FUNCTION "CICLO FORMAZIONE PACCHI" : VOID
TITLE =CICLO AUTOMATICO FORMAZIONE PACCHI
VERSION : 0.1

BEGIN
NETWORK
TITLE =START CICLO
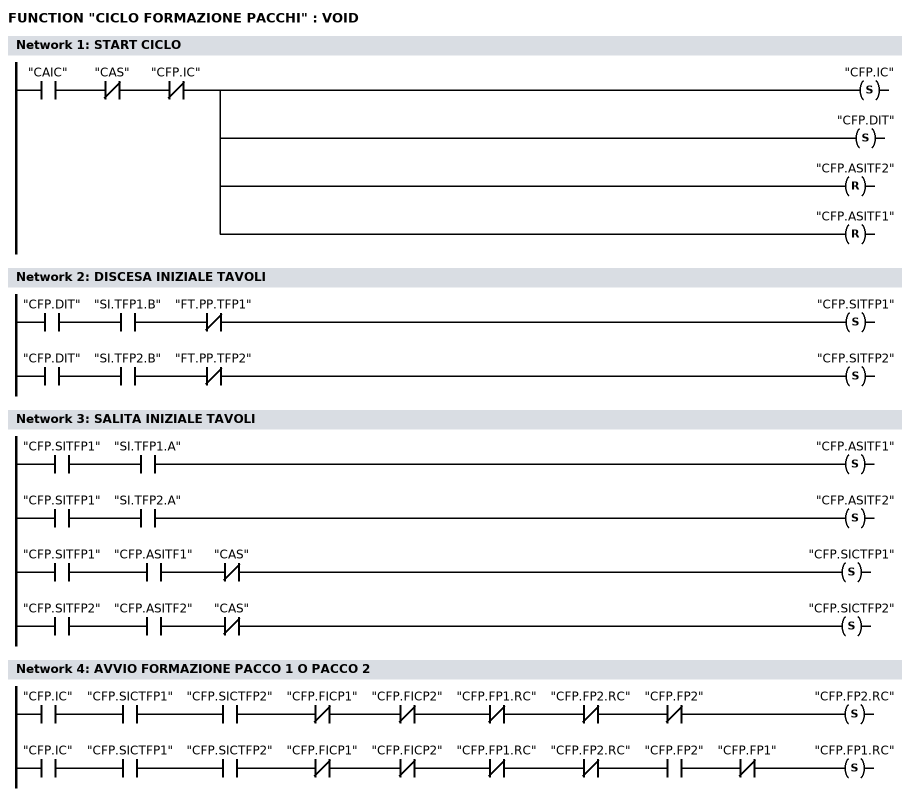
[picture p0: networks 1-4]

      U     "CAIC";
      UN    "CAS";
      UN    "CFP.IC";
      S     "CFP.IC";
      S     "CFP.DIT";
      R     "CFP.ASITF2";
      R     "CFP.ASITF1";
NETWORK
TITLE =DISCESA INIZIALE TAVOLI

      U     "CFP.DIT";
      U     "SI.TFP1.B";
      UN    "FT.PP.TFP1";
      S     "CFP.SITFP1";
//-----------------------------
      U     "CFP.DIT";
      U     "SI.TFP2.B";
      UN    "FT.PP.TFP2";
      S     "CFP.SITFP2";

NETWORK
TITLE =SALITA INIZIALE TAVOLI

      U     "CFP.SITFP1";
      U     "SI.TFP1.A";
      S     "CFP.ASITF1";
//---------------------------
      U     "CFP.SITFP1";
      U     "SI.TFP2.A";
      S     "CFP.ASITF2";
//====================================
      U     "CFP.SITFP1";
      U     "CFP.ASITF1";
      UN    "CAS";
      S     "CFP.SICTFP1";
//====================================
      U     "CFP.SITFP2";
      U     "CFP.ASITF2";
      UN    "CAS";
      S     "CFP.SICTFP2";

NETWORK
TITLE =AVVIO FORMAZIONE PACCO 1 O PACCO 2

      U     "CFP.IC";
      U     "CFP.SICTFP1";
      U     "CFP.SICTFP2";
      UN    "CFP.FICP1";
      UN    "CFP.FICP2";
      UN    "CFP.FP1.RC";
      UN    "CFP.FP2.RC";
      UN    "CFP.FP2";
      S     "CFP.FP2.RC";
//-----------------------
      U     "CFP.IC";
      U     "CFP.SICTFP1";
      U     "CFP.SICTFP2";
      UN    "CFP.FICP1";
      UN    "CFP.FICP2";
      UN    "CFP.FP1.RC";
      UN    "CFP.FP2.RC";
      U     "CFP.FP2";
      UN    "CFP.FP1";
      S     "CFP.FP1.RC";

NETWORK
TITLE =FORMAZIONE PACCO 2

//____________________________________
//      Inizio ciclo
//____________________________________
      U     "CFP.FP2.RC";
      UN    "CFP.FP2";
      S     "CFP.FP2";
      S     "CFP.FICP2";
      R     "CNP.FP2";
      R     "CFP.FP2.RC";
//____________________________________
//      Inibizione discesa tavolo
//____________________________________
      U     "CFP.FP2";
      U     "CFP.FICP2";
      U     "SI.PCA";
      S     "CFP.IDTF2";
      S     "CFP.CAP2";
//____________________________________
//      Discesa tavolo
//____________________________________
      U     "CFP.FP2";
      U     "CFP.FICP2";
      U     "FT.CLP.FP2";
      UN    "CFP.IDTF2";
      UN    "CAS";
      U     "SM.AFA.P2";
      U     "SM.ALSA.P2";
      U     "SM.ALDA.P2";
      =     "CFP.DTF2";
//____________________________________
//      Conteggio piastre
//____________________________________
      U     "CFP.FP2";
      U     "CFP.FICP2";
      UN    "CFP.BPIASP2";
      U     "CFP.MPCP";
      UN    "CFP.BP2F";
      FP    "CFP.ACPP2";
      ZV    "CNP.FP2";
//____________________________________
//      Allineamento pacco
//____________________________________
      U     "CFP.FP2";
      U     "CFP.FICP2";
      U     "CFP.CAP2";
      U     "FN.SI.PCP.FP2";
      R     "CFP.CAP2";
//-----
      U     "CFP.FP2";
      U     "CFP.FICP2";
      UN    "CFP.CAP2";
      U     "SM.AFA.P2";
      U     "SM.ALSA.P2";
      U     "SM.ALDA.P2";
      L     "DB TEMPI".T_RPPSTFP2;
      SE    "T.RPPSTFP2";
//------------------------------------
      U     "T.RPPSTFP2";
      R     "CFP.IDTF2";
//____________________________________
//      Controllo pacco formato
//____________________________________
      U     "CFP.FP2";
      U     "CFP.FICP2";
      U     "CFP.BPIASP2";
      U     "FN.SI.PCP.FP1";
      R     "CFP.BPIASP2";
      R     "CNP.FP2";
//------------------------------------
      L     "CNP.FP2";
      L     2;
      *I    ;
      L     "DB DATI".NPPP;
      >=I   ;
      U     "CFP.FP2";
      U     "CFP.FICP2";
      U     "FN.SI.PCP.FP1";
      S     "CFP.BP2F";
      S     "CFP.FP1.RC";
      S     "CFP.BPIASP2";
//____________________________________
//      Attesa per discesa finale
//____________________________________
      U     "CFP.FP2";
      U     "CFP.BP2F";
      UN    "CFP.BPIASP2";
      UN    "CFP.IDTF2";
      UN    "CFP.DFTF2";
      UN    "CFP.ASP2";
      UN    "CFP.STF2";
      S     "CFP.DFTF2";
      S     "CFP.BRUAP2";
      R     "CFP.FICP2";
//____________________________________
//      Ultimo allineamento
//____________________________________
      U     "CFP.BRUAP2";
      UN    "CFP.BPIASP2";
      L     "DB TEMPI".T_DPAFP2;
      SE    "T.DPAFP2";
//------------------------------------
      U     "T.DPAFP2";
      UN    "SM.ALDA.P2";
      UN    "SM.ALSA.P2";
      UN    "SM.AFA.P2";
      S     "CFP.AUAP2";
//------------------------------------
      U     "T.DPAFP2";
      U     "CFP.AUAP2";
      U     "SM.ALDA.P2";
      U     "SM.ALSA.P2";
      U     "SM.AFA.P2";
      R     "CFP.BRUAP2";
      R     "CFP.AUAP2";
//____________________________________
//      Discesa finale tavolo
//____________________________________
      U     "CFP.DFTF2";
      U     "SI.TFP2.IA";
      S     "CFP.ASP2";
      R     "CFP.DFTF2";
//____________________________________
//      Attesa scarico pacco per salita
//____________________________________
      U     "CFP.ASP2";
      U     "CCUG.CS2.GS";
      S     "CFP.STF2";
      R     "CFP.ASP2";
//____________________________________
//      Salita finale tavolo
//____________________________________
      U     "CFP.STF2";
      U     "SI.TFP2.A";
      R     "CFP.STF2";
      R     "CFP.FP2";
      R     "CFP.BP2F";

NETWORK
TITLE =FORMAZIONE PACCO 1

//____________________________________
//      Inizio ciclo
//____________________________________
      U     "CFP.FP1.RC";
      UN    "CFP.FP1";
      S     "CFP.FP1";
      S     "CFP.FICP1";
      R     "CNP.FP1";
      R     "CFP.FP1.RC";
//____________________________________
//      Inibizione discesa tavolo
//____________________________________
      U     "CFP.FP1";
      U     "CFP.FICP1";
      U     "SI.PCA";
      S     "CFP.IDTF1";
      S     "CFP.CAP1";
//____________________________________
//      Discesa tavolo
//____________________________________
      U     "CFP.FP1";
      U     "CFP.FICP1";
      U     "FT.CLP.FP1";
      UN    "CFP.IDTF1";
      UN    "CAS";
      U     "SM.AFA.P1";
      U     "SM.ALSA.P1";
      U     "SM.ALDA.P1";
      =     "CFP.DTF1";
//____________________________________
//      Conteggio piastre
//____________________________________
      U     "CFP.FP1";
      U     "CFP.FICP1";
      UN    "CFP.BP1F";
      U     "CFP.MPCP";
      FP    "CFP.ACPP1";
      ZV    "CNP.FP1";
//____________________________________
//      Allineamento pacco
//____________________________________
      U     "CFP.FP1";
      U     "CFP.FICP1";
      U     "CFP.CAP1";
      U     "FN.SI.PCP.FP1";
      R     "CFP.CAP1";
//-----
      U     "CFP.FP1";
      U     "CFP.FICP1";
      UN    "CFP.CAP1";
      U     "SM.AFA.P1";
      U     "SM.ALSA.P1";
      U     "SM.ALDA.P1";
      L     "DB TEMPI".T_RPPSTFP1;
      SE    "T.RPPSTFP1";
//------------------------------------
      U     "T.RPPSTFP1";
      R     "CFP.IDTF1";
//____________________________________
//      Controllo pacco formato
//____________________________________
      L     "CNP.FP1";
      L     2;
      *I    ;
      L     "DB DATI".NPPP;
      >=I   ;
      U     "CFP.FP1";
      U     "CFP.FICP1";
      U     "FN.SI.PCP.FP2";
      S     "CFP.BP1F";
      S     "CFP.FP2.RC";
//____________________________________
//      Attesa per discesa finale
//____________________________________
      U     "CFP.FP1";
      U     "CFP.BP1F";
      UN    "CFP.IDTF1";
      UN    "CFP.DFTF1";
      UN    "CFP.ASP1";
      UN    "CFP.STF1";
      S     "CFP.DFTF1";
      S     "CFP.BRUAP1";
      R     "CFP.FICP1";
//____________________________________
//      Ultimo allineamento
//____________________________________
      U     "CFP.BRUAP1";
      UN    "CFP.BPIASP1";
      L     "DB TEMPI".T_DPAFP1;
      SE    "T.DPAFP1";
//------------------------------------
      U     "T.DPAFP1";
      UN    "SM.ALDA.P1";
      UN    "SM.ALSA.P1";
      UN    "SM.AFA.P1";
      S     "CFP.AUAP1";
//------------------------------------
      U     "T.DPAFP1";
      U     "CFP.AUAP1";
      U     "SM.ALDA.P1";
      U     "SM.ALSA.P1";
      U     "SM.AFA.P1";
      R     "CFP.BRUAP1";
      R     "CFP.AUAP1";
//____________________________________
//      Discesa finale tavolo
//____________________________________
      U     "CFP.DFTF1";
      U     "SI.TFP1.IA";
      S     "CFP.ASP1";
      R     "CFP.DFTF1";
//____________________________________
//      Attesa scarico pacco per salita
//____________________________________
      U     "CFP.ASP1";
      U     "CCUG.CS1.GS";
      S     "CFP.STF1";
      R     "CFP.ASP1";
//____________________________________
//      Salita finale tavolo
//____________________________________
      U     "CFP.STF1";
      U     "SI.TFP1.A";
      R     "CFP.STF1";
      R     "CFP.FP1";
      R     "CFP.BP1F";

NETWORK
TITLE =MEMORIA PER CONTEGGIO PIASTRE
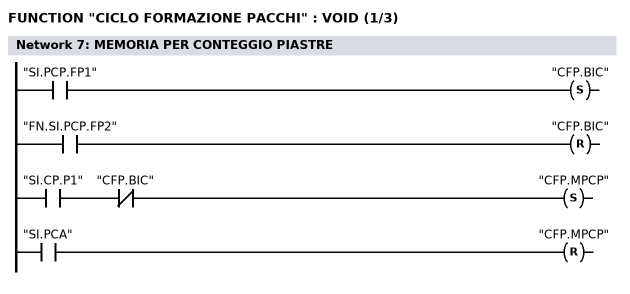
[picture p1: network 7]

      U     "SI.PCP.FP1";
      S     "CFP.BIC";
//----------------------------------
      U     "FN.SI.PCP.FP2";
      R     "CFP.BIC";
//==================================
      U     "SI.CP.P1";
      UN    "CFP.BIC";
      S     "CFP.MPCP";
//----------------------------------
      U     "SI.PCA";
      R     "CFP.MPCP";

NETWORK
TITLE =RICHIESTA COMANDO USCITE
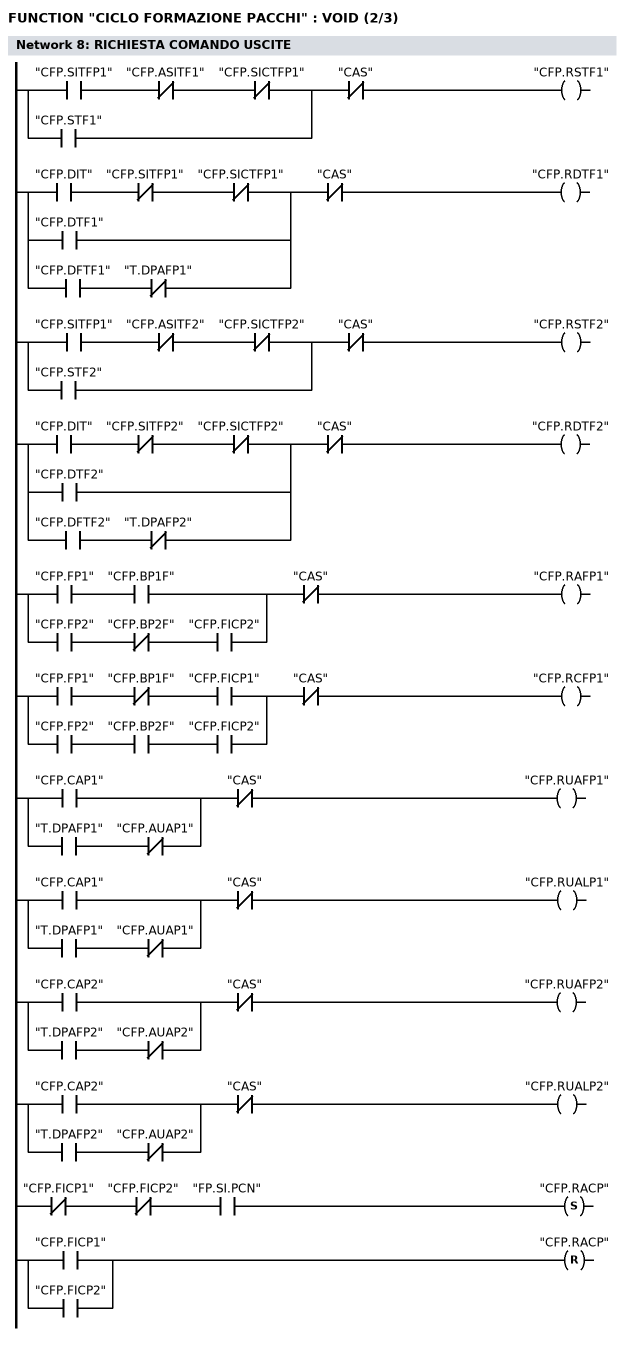
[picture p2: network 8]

//    SALITA TAVOLO FORMAZIONE 1
//_____________________________________
      U(    ;
      U     "CFP.SITFP1";
      UN    "CFP.ASITF1";
      UN    "CFP.SICTFP1";
      O     ;
      U     "CFP.STF1";
      )     ;
      UN    "CAS";
      =     "CFP.RSTF1";
//=====================================
//    DISCESA TAVOLO FORMAZIONE 1
//_____________________________________
      U(    ;
      U     "CFP.DIT";
      UN    "CFP.SITFP1";
      UN    "CFP.SICTFP1";
      O     ;
      U     "CFP.DTF1";
      O     ;
      U     "CFP.DFTF1";
      UN    "T.DPAFP1";
      )     ;
      UN    "CAS";
      =     "CFP.RDTF1";
//=====================================
//    SALITA TAVOLO FORMAZIONE 2
//_____________________________________
      U(    ;
      U     "CFP.SITFP1";
      UN    "CFP.ASITF2";
      UN    "CFP.SICTFP2";
      O     ;
      U     "CFP.STF2";
      )     ;
      UN    "CAS";
      =     "CFP.RSTF2";
//=====================================
//    DISCESA TAVOLO FORMAZIONE 2
//_____________________________________
      U(    ;
      U     "CFP.DIT";
      UN    "CFP.SITFP2";
      UN    "CFP.SICTFP2";
      O     ;
      U     "CFP.DTF2";
      O     ;
      U     "CFP.DFTF2";
      UN    "T.DPAFP2";
      )     ;
      UN    "CAS";
      =     "CFP.RDTF2";
//=====================================
//    APERTURA FERMO PACCO 1
//_____________________________________
      U(    ;
      U     "CFP.FP1";
      U     "CFP.BP1F";
      O     ;
      U     "CFP.FP2";
      UN    "CFP.BP2F";
      U     "CFP.FICP2";
      )     ;
      UN    "CAS";
      =     "CFP.RAFP1";
//=====================================
//    CHIUSURA FERMO PACCO 1
//_____________________________________
      U(    ;
      U     "CFP.FP1";
      UN    "CFP.BP1F";
      U     "CFP.FICP1";
      O     ;
      U     "CFP.FP2";
      U     "CFP.BP2F";
      U     "CFP.FICP2";
      )     ;
      UN    "CAS";
      =     "CFP.RCFP1";
//=====================================
//    USCITA ALLINEATORE FRONTALE PACCO 1
//_____________________________________
      U(    ;
      U     "CFP.CAP1";
      O     ;
      U     "T.DPAFP1";
      UN    "CFP.AUAP1";
      )     ;
      UN    "CAS";
      =     "CFP.RUAFP1";
//=====================================
//    USCITA ALLINEATORI LATERALI PACCO 1
//_____________________________________
      U(    ;
      U     "CFP.CAP1";
      O     ;
      U     "T.DPAFP1";
      UN    "CFP.AUAP1";
      )     ;
      UN    "CAS";
      =     "CFP.RUALP1";
//=====================================
//    USCITA ALLINEATORE FRONTALE PACCO 2
//_____________________________________
      U(    ;
      U     "CFP.CAP2";
      O     ;
      U     "T.DPAFP2";
      UN    "CFP.AUAP2";
      )     ;
      UN    "CAS";
      =     "CFP.RUAFP2";
//=====================================
//    USCITA ALLINEATORI LATERALI PACCO 2
//_____________________________________
      U(    ;
      U     "CFP.CAP2";
      O     ;
      U     "T.DPAFP2";
      UN    "CFP.AUAP2";
      )     ;
      UN    "CAS";
      =     "CFP.RUALP2";
//=====================================
//    RICHIESTA ARRESTO CATENE PRINCIPALI
//_____________________________________
      UN    "CFP.FICP1";
      UN    "CFP.FICP2";
      U     "FP.SI.PCN";
      S     "CFP.RACP";
//------------------------------
      O     "CFP.FICP1";
      O     "CFP.FICP2";
      R     "CFP.RACP";

NETWORK
TITLE =RESET CICLO
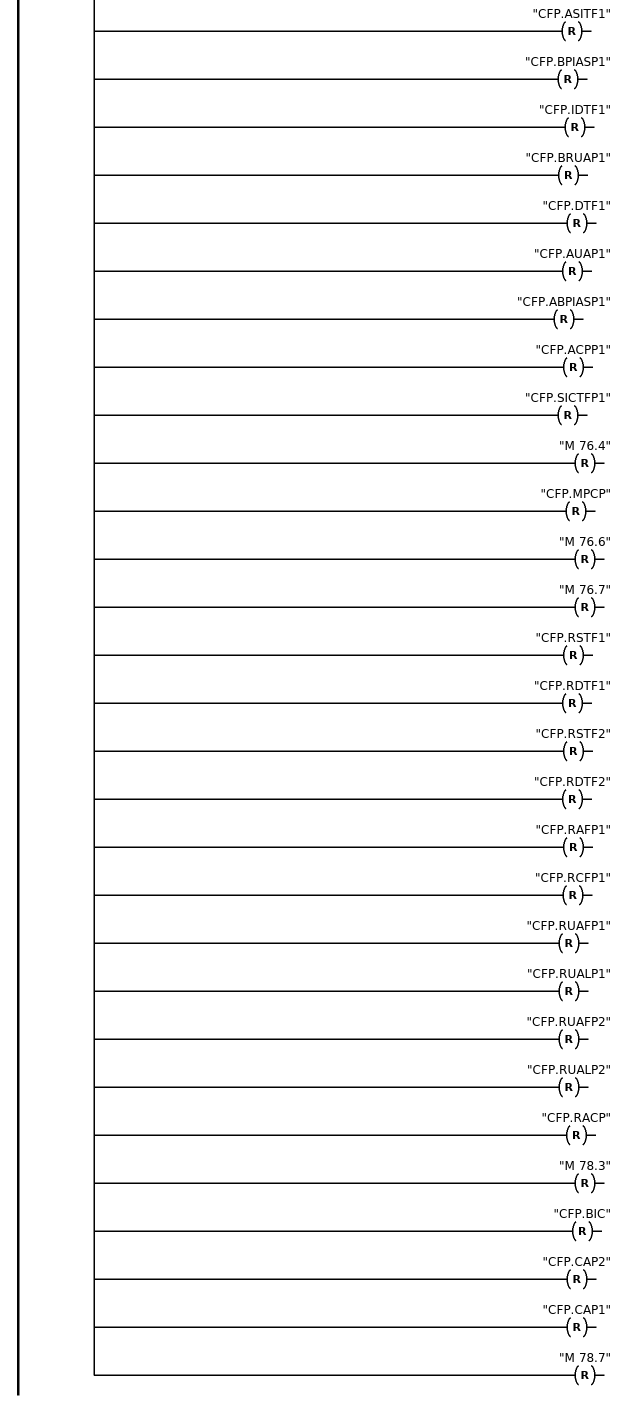
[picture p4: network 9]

      U     "TRT";
//      O     "PL.S.PR"
      R     "CFP.IC";
      R     "CFP.DIT";
      R     "CFP.SITFP1";
      R     "CFP.SITFP2";
      R     "CFP.FP2.RC";
      R     "CFP.FP2";
      R     "CFP.FICP2";
      R     "CFP.BP2F";
      R     "CFP.DFTF2";
      R     "CFP.ASP2";
      R     "CFP.STF2";
      R     "CFP.ASITF2";
      R     "CFP.BPIASP2";
      R     "CFP.IDTF2";
      R     "CFP.BRUAP2";
      R     "CFP.DTF2";
      R     "CFP.AUAP2";
      R     "CFP.ABPIASP2";
      R     "CFP.ACPP2";
      R     "CFP.SICTFP2";
      R     "CFP.FP1.RC";
      R     "CFP.FP1";
      R     "CFP.FICP1";
      R     "CFP.BP1F";
      R     "CFP.DFTF1";
      R     "CFP.ASP1";
      R     "CFP.STF1";
      R     "CFP.ASITF1";
      R     "CFP.BPIASP1";
      R     "CFP.IDTF1";
      R     "CFP.BRUAP1";
      R     "CFP.DTF1";
      R     "CFP.AUAP1";
      R     "CFP.ABPIASP1";
      R     "CFP.ACPP1";
      R     "CFP.SICTFP1";
      R     "M      76.4";
      R     "CFP.MPCP";
      R     "M      76.6";
      R     "M      76.7";
      R     "CFP.RSTF1";
      R     "CFP.RDTF1";
      R     "CFP.RSTF2";
      R     "CFP.RDTF2";
      R     "CFP.RAFP1";
      R     "CFP.RCFP1";
      R     "CFP.RUAFP1";
      R     "CFP.RUALP1";
      R     "CFP.RUAFP2";
      R     "CFP.RUALP2";
      R     "CFP.RACP";
      R     "M      78.3";
      R     "CFP.BIC";
      R     "CFP.CAP2";
      R     "CFP.CAP1";
      R     "M      78.7";

END_FUNCTION

